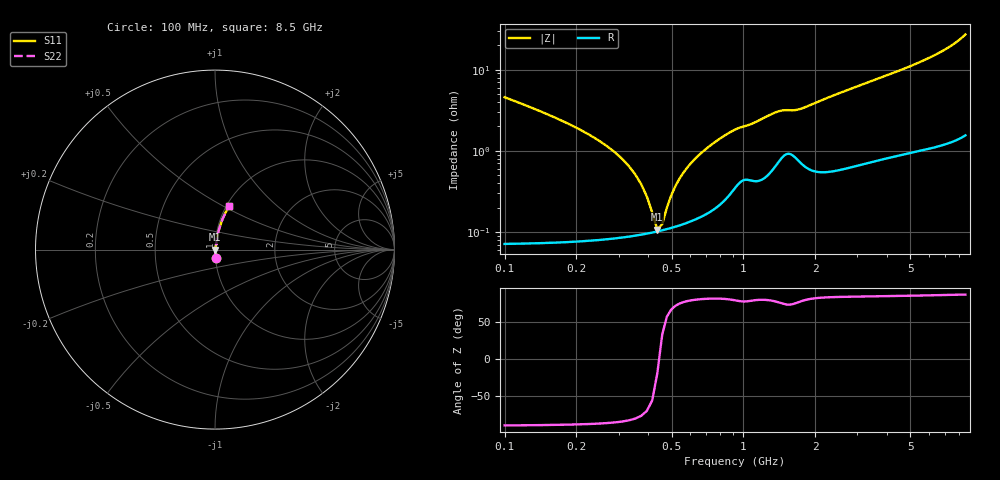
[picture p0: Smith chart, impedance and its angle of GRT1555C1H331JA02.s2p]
!Murata Part Number: GRT1555C1H331JA02
!These Parameters are Measured in Series Mode Connection
!Data Generated on Jun 19, 2026
!  o--ll--o
!Port1  Port2
!  o------o
!Operation Temp=25[degC], DC Bias Voltage=0[V]
!Freq. Start=100[MHz] Stop=9[GHz] 401[Steps]
# Hz S RI R 50
!Freq.(Hz) S11(Real) S11(Imag) S21(Real) S21(Imag) S12(Real) S12(Imag) S22(Real) S22(Imag)
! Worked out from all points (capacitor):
!   401 points, 100 MHz to 8.5 GHz, reference 50 ohm
!   read as one part in series: C = 330 pF near 142 MHz
!   lowest |Z| = 108 mohm at 436 MHz (marker M1)
!   series resonance near 443.1 MHz, so ESL is about 390 pH
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1e8  0.0028 -0.0456  0.9972 0.0456  0.9972 0.0456  0.0028 -0.0456
1.42e8  0.00166 -0.0304  0.9983 0.0304  0.9983 0.0304  0.00166 -0.0304
3.1e8  0.000917 -0.00795  0.9991 0.00795  0.9991 0.00795  0.000917 -0.00795
3.52e8  0.000927 -0.00506  0.9991 0.00506  0.9991 0.00506  0.000927 -0.00506
4.15e8  0.000986 -0.00143  0.999 0.00143  0.999 0.00143  0.000986 -0.00143
4.36e8  0.00102 -0.000349  0.999 0.000349  0.999 0.000349  0.00102 -0.000349
4.57e8  0.00105 0.00068  0.999 -0.00068  0.999 -0.00068  0.00105 0.00068
4.78e8  0.00109 0.00167  0.9989 -0.00167  0.9989 -0.00167  0.00109 0.00167
5.41e8  0.00123 0.00442  0.9988 -0.00442  0.9988 -0.00442  0.00123 0.00442
5.83e8  0.00134 0.00612  0.9987 -0.00612  0.9987 -0.00612  0.00134 0.00612
6.67e8  0.00163 0.00931  0.9984 -0.00931  0.9984 -0.00931  0.00163 0.00931
7.72e8  0.00218 0.0131  0.9978 -0.0131  0.9978 -0.0131  0.00218 0.0131
9.61e8  0.00434 0.0186  0.9957 -0.0186  0.9957 -0.0186  0.00434 0.0186
1.339e9  0.00683 0.0282  0.9932 -0.0282  0.9932 -0.0282  0.00683 0.0282
1.507e9  0.00986 0.0299  0.9901 -0.0299  0.9901 -0.0299  0.00986 0.0299
1.717e9  0.00827 0.0313  0.9917 -0.0313  0.9917 -0.0313  0.00827 0.0313
2.284e9  0.00752 0.0449  0.9925 -0.0449  0.9925 -0.0449  0.00752 0.0449
2.914e9  0.0099 0.0591  0.9901 -0.0591  0.9901 -0.0591  0.0099 0.0591
4.3e9  0.0167 0.0899  0.9833 -0.0899  0.9833 -0.0899  0.0167 0.0899
5.707e9  0.0264 0.1257  0.9736 -0.1257  0.9736 -0.1257  0.0264 0.1257
7.114e9  0.0432 0.1726  0.9568 -0.1726  0.9568 -0.1726  0.0432 0.1726
8.5e9  0.0807 0.2453  0.9193 -0.2453  0.9193 -0.2453  0.0807 0.2453
